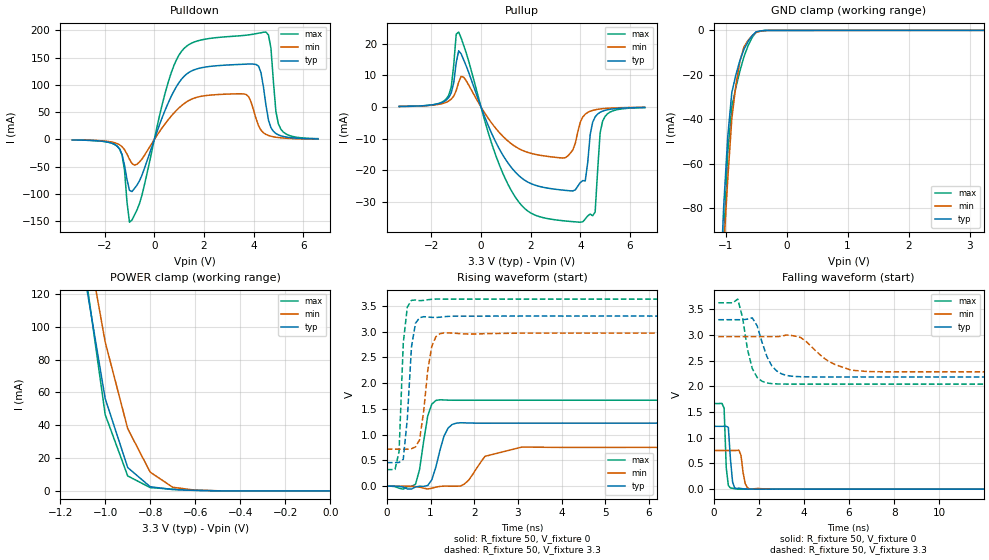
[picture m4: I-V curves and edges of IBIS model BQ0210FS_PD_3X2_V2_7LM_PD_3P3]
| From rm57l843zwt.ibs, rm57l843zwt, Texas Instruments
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|   Model Cell BQ0210FS_PD_3X2_V2_7LM_PD_3P3
|BQ0210FS_PD_3X2_V2_7LM_PD_3P3
[Model]   BQ0210FS_PD_3X2_V2_7LM_PD_3P3
Model_type   I/O
Polarity   Non-Inverting
Enable   Active-Low
Vinl =  1.15
Vinh =  1.55
Cref =  15.0001pF
Rref =  101.0000M
Vref =  0V
Vmeas =  1.65
C_comp   1.2p   1.2p   1.2p
[Model Spec]
Vinl   1.15   1.02   1.28
Vinh   1.55   1.45   1.65
[Temperature Range]   25   155   -40
[Voltage Range]   3.3   2.97   3.63
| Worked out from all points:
|   slope of the pulldown table from 0 to 0.495 V, typ, clamps not added: 8.21 ohm
|   slope of the pullup table from 0 to 0.495 V, typ, clamps not added: 52.1 ohm
|   GND clamp passes 1 mA (typ) near -0.51 V on its own axis
|   POWER clamp passes 1 mA (typ) near -0.71 V on its own axis
|   rising waveform, R_fixture 50, V_fixture 0: 20-80 % time 238ps typ, 454ps min, 180ps max; typ from 0 V to 1.22 V
|   rising waveform, R_fixture 50, V_fixture 3.3: 20-80 % time 135ps typ, 196ps min, 107ps max; typ from 0.458 V to 3.3 V
|   falling waveform, R_fixture 50, V_fixture 0: 20-80 % time 132ps typ, 153ps min, 97.7ps max; typ from 1.22 V to 0 V
|   falling waveform, R_fixture 50, V_fixture 3.3: 20-80 % time 29.5ns typ, 30.7ns min, 18.4ns max; typ from 3.3 V to 0.465 V
[POWER_clamp]
|   voltage   I(typ)   I(min)   I(max)
-3.3V     2.37A      2.626A     3.145A
-1.1V     138.4mA    167.6mA    144.8mA
-1.067V   111mA      142mA      112mA
-1.033V   83.64mA    116.3mA    79.25mA
-1V       56.26mA    90.72mA    46.5mA
-900mV    14.24mA    37.93mA    9.136mA
-800mV    2.556mA    11.42mA    2.04mA
-700mV    826.2uA    2.23mA     1.064mA
-600mV    300.3uA    462.9uA    402.5uA
-500mV    67.45uA    107.7uA    90.06uA
0V        19.75uA    8.573uA    38.26uA
[Pulldown]
|   voltage   I(typ)   I(min)   I(max)
-3.3V     -899.6uA   -820.6uA   -837.7uA
-1.4V     -17.27mA   -9.734mA   -17.51mA
-1.2V     -47.62mA   -18.77mA   -56.87mA
-1V       -93.34mA   -36.32mA   -151.7mA
1.1V      110.9mA    62.27mA    162mA
3.6V      138mA      83.62mA    190.9mA
4.1V      137.6mA    38.13mA    194.2mA
4.5V      62.69mA    9.297mA    197.1mA
4.7V      21.72mA    5.946mA    167.7mA
4.9V      10.98mA    4.145mA    51.34mA
5.1V      6.781mA    3.055mA    18.84mA
6.6V      1.042mA    806uA      1.545mA
[Pullup]
|   voltage   I(typ)   I(min)   I(max)
-3.3V     154uA      152.3uA    178.5uA
-1.4V     2.171mA    1.484mA    2.544mA
-900mV    17.81mA    7.857mA    23.72mA
500mV     -9.587mA   -5.844mA   -13.22mA
1.4V      -20.78mA   -12.62mA   -28.76mA
3.4V      -26.42mA   -16.07mA   -36.11mA
4V        -23.95mA   -4.859mA   -36.5mA
4.2V      -23.43mA   -2.288mA   -35.5mA
4.6V      -3.136mA   -899.4uA   -33.27mA
4.8V      -1.694mA   -637.7uA   -8.23mA
5V        -1.071mA   -474.1uA   -2.98mA
6.6V      -155uA     -124.4uA   -196.9uA
[GND_clamp]
|   voltage   I(typ)   I(min)   I(max)
-3.3V     -1.949A    -1.625A    -3.258A
-1.1V     -122.2mA   -133.9mA   -153mA
-1.033V   -79.16mA   -98.31mA   -94.35mA
-966.7mV  -47.75mA   -66.92mA   -54.8mA
-900mV    -27.96mA   -39.72mA   -34.3mA
-833.3mV  -19.96mA   -24.61mA   -25.7mA
-766.7mV  -13.47mA   -13.82mA   -18.19mA
-700mV    -8.475mA   -7.367mA   -11.76mA
-566.7mV  -2.401mA   -2.353mA   -3.191mA
-500mV    -637.2uA   -903uA     -737.8uA
-300mV    -7.458uA   -14.4uA    -10.67uA
3.233V    19.75uA    9.636uA    38.26uA
[Ramp]
| variable   typ   min   max
dV/dt_f   1.749279/29.50598n   0.5677296/0.3497717n   2.039724/18.38714n
dV/dt_r  0.7830634/0.2506344n   0.49096/0.4107292n   1.052126/0.1907457n
R_load = 50
[Rising Waveform]
R_fixture = 50
V_fixture = 0
V_fixture_min = 0
V_fixture_max = 0
|   time   V(typ)   V(min)   V(max)
0s        -5.649uV   -3.893uV   -12.5uV
656ps     -14.37mV   -7.691mV   38.47mV
748ps     -1.46mV    -18.27mV   318.9mV
936ps     13.96mV    -54.1mV    1.363V
1.216ns   698.1mV    -3.534mV   1.676V
1.496ns   1.198V     -641uV     1.668V
1.872ns   1.226V     117.5mV    1.667V
2.244ns   1.222V     578.9mV    1.668V
3.092ns   1.223V     759.4mV    1.668V
35.52ns   1.224V     752.9mV    1.668V
[Rising Waveform]
R_fixture = 50
V_fixture = 3.3
V_fixture_min = 2.97
V_fixture_max = 3.63
|   time   V(typ)   V(min)   V(max)
0s        457.5mV    717.2mV    321.6mV
188ps     457.3mV    717.3mV    326.6mV
280ps     460.4mV    717.2mV    673.2mV
376ps     522.9mV    716.7mV    2.775V
468ps     1.302V     716.9mV    3.473V
564ps     2.702V     727.6mV    3.605V
748ps     3.267V     896.7mV    3.599V
1.028ns   3.275V     2.712V     3.626V
1.308ns   3.287V     2.972V     3.629V
35.52ns   3.3V       2.97V      3.629V
[Falling Waveform]
R_fixture = 50
V_fixture = 0
V_fixture_min = 0
V_fixture_max = 0
|   time   V(typ)   V(min)   V(max)
0s        1.224V     752.9mV    1.668V
468ps     1.224V     752.9mV    1.577V
564ps     1.224V     752.9mV    414.8mV
656ps     1.204V     752.9mV    72.02mV
844ps     141.2mV    753.2mV    17.48mV
1.028ns   13.33mV    753.5mV    2.829mV
1.216ns   13.86mV    659.3mV    783uV
1.404ns   3.452mV    105.7mV    991.6uV
1.684ns   591.3uV    257uV      796.4uV
35.52ns   158.2uV    1.962uV    1.899uV
[Falling Waveform]
R_fixture = 50
V_fixture = 3.3
V_fixture_min = 2.97
V_fixture_max = 3.63
|   time   V(typ)   V(min)   V(max)
212ps     3.3V       2.97V      3.629V
1.072ns   3.299V     2.97V      3.702V
1.716ns   3.335V     2.97V      2.349V
2.364ns   2.582V     2.97V      2.068V
18.34ns   2.185V     2.285V     2.05V
20.97ns   2.185V     2.285V     477mV
29.3ns    2.186V     2.285V     345mV
34.98ns   551.4mV    2.285V     344.8mV
36.08ns   525.4mV    755.6mV    344.8mV
36.96ns   465.4mV    755.6mV    344.8mV
